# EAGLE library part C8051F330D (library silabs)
8kB ILP Flash MCU Family Source: www.silabs.com .. C8051F33x.pdf
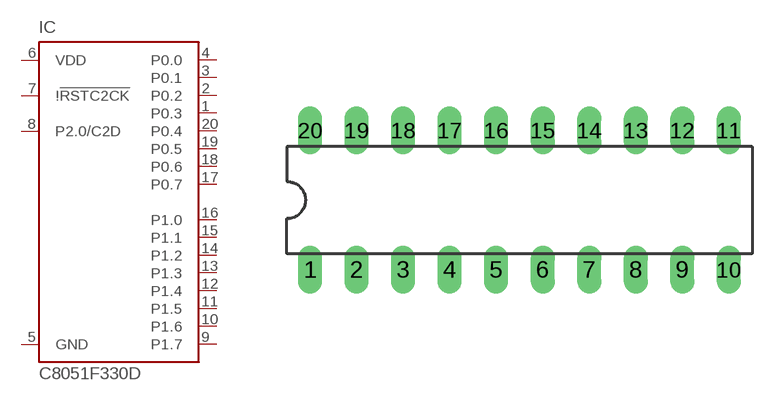
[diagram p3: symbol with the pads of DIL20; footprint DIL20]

Designator prefix IC

## C8051F330D (OC_FARNELL: unknown; OC_NEWARK: unknown)  [DIL20]
1  P0.3
2  P0.2
3  P0.1
4  P0.0
5  GND  pwr
6  VDD  pwr
7  !!RSTC2CK  in
8  P2.0/C2D
9  P1.7
10  P1.6
11  P1.5
12  P1.4
13  P1.3
14  P1.2
15  P1.1
16  P1.0
17  P0.7
18  P0.6
19  P0.5
20  P0.4

## Footprint DIL20 (pad centres in mm)
Dual In Line Package
drill 0.813 long: 1 -11.43,-3.81; 2 -8.89,-3.81; 3 -6.35,-3.81; 4 -3.81,-3.81; 5 -1.27,-3.81; 6 1.27,-3.81; 7 3.81,-3.81; 8 6.35,-3.81; 9 8.89,-3.81; 10 11.43,-3.81; 11 11.43,3.81; 12 8.89,3.81; 13 6.35,3.81; 14 3.81,3.81; 15 1.27,3.81; 16 -1.27,3.81; 17 -3.81,3.81; 18 -6.35,3.81; 19 -8.89,3.81; 20 -11.43,3.81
